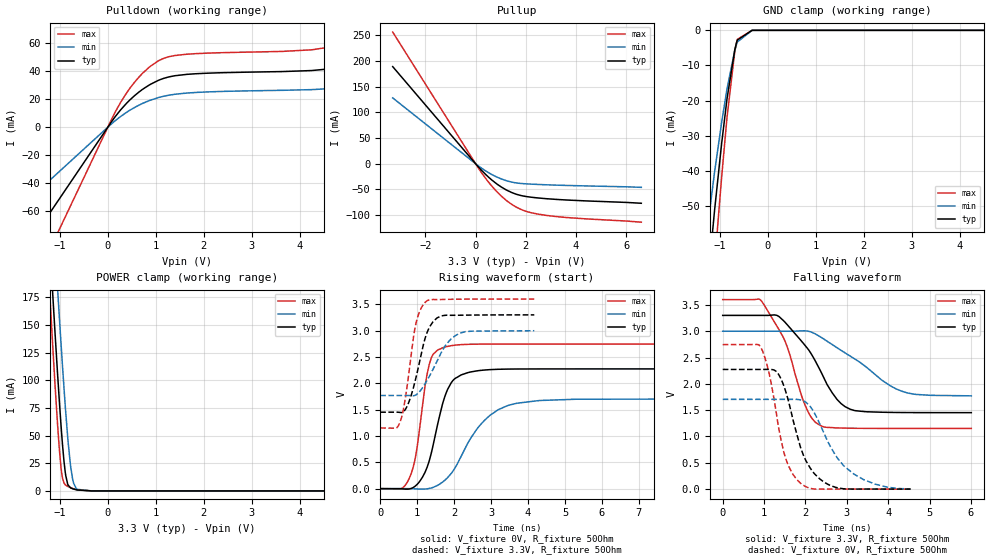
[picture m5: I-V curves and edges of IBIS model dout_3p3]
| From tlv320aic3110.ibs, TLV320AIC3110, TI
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|   dout_3p3 Model
[Model]   dout_3p3
Model_type   3-state
Polarity   Non-Inverting
Vmeas = 1.65
Vref = 0
Cref = 10pF
Rref = 50
|   typ   min   max
|   (nom PVT)   (fast PVT)   (slow PVT)
C_comp   1.577e-12   1.531e-12   1.633e-12
| Where nom  PVT is Nominal Process, 3.3V, 27C
|   Fast PVT is Strong Process,  3.6V, -40C
|   Slow PVT is Weak Process,   3V, 125C
[Voltage Range]   3.3   3   3.6
|Junction Temperature
[Temperature Range]   27   125   -40
[Pullup Reference]   3.3   3   3.6
[Pulldown Reference]   0   0   0
[Power Clamp Reference]   3.3   3   3.6
[GND Clamp Reference]   0   0   0
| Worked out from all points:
|   slope of the pulldown table from 0 to 0.495 V, typ, clamps not added: 24.1 ohm
|   slope of the pullup table from 0 to 0.495 V, typ, clamps not added: 19.6 ohm
|   POWER clamp passes 1 mA (typ) near -0.65 V on its own axis
|   falling waveform, V_fixture 3.3V, R_fixture 50Ohm: 20-80 % time 881ps typ, 1.32ns min, 668ps max; typ from 3.3 V to 1.45 V
|   rising waveform, V_fixture 0V, R_fixture 50Ohm: 20-80 % time 494ps typ, 951ps min, 336ps max; typ from 0 V to 2.27 V
|   rising waveform, V_fixture 3.3V, R_fixture 50Ohm: 20-80 % time 392ps typ, 569ps min, 297ps max; typ from 1.45 V to 3.3 V
|   falling waveform, V_fixture 0V, R_fixture 50Ohm: 20-80 % time 536ps typ, 810ps min, 414ps max; typ from 2.27 V to 0 V
[Pulldown]
|   Voltage   I(typ)   I(min)   I(max)
-3.3V     -167.2mA   -103.4mA   -238.3mA
-142.8mV  -7.234mA   -4.473mA   -10.31mA
153mV     7.459mA    4.581mA    10.75mA
462mV     19.5mA     12.14mA    27.88mA
855mV     29.92mA    18.83mA    42.57mA
1.164V    34.82mA    22.06mA    49.12mA
1.827V    38.11mA    24.74mA    52.46mA
4.713V    41.96mA    27.72mA    57.69mA
5.409V    48.18mA    31.48mA    67.5mA
5.732V    53.68mA    34.86mA    76.04mA
6.33V     70.28mA    45.19mA    101.5mA
6.6V      81.15mA    52.04mA    118mA
[GND Clamp]
|   Voltage   I(typ)   I(min)   I(max)
-3.3V     -1.792A    -1.545A    -1.979A
-1.482V   -105.6mA   -80.57mA   -134.7mA
-1.119V   -52.39mA   -41.19mA   -68.09mA
-1.104V   -50.35mA   -39.68mA   -65.46mA
-966.9mV  -32.64mA   -26.54mA   -42.36mA
-851.4mV  -19.49mA   -16.66mA   -24.78mA
-690mV    -5.595mA   -5.789mA   -6.089mA
-660mV    -3.881mA   -4.332mA   -3.916mA
-636mV    -2.764mA   -3.329mA   -2.575mA
-330mV    -1.038uA   -9.723uA   -110.9nA
6.6V      0A         0A         0A
[Pullup]
|   Voltage   I(typ)   I(min)   I(max)
-3.3V     189.2mA    128.2mA    256.5mA
181.2mV   -9.972mA   -6.723mA   -13.56mA
492mV     -25.14mA   -16.79mA   -34.41mA
786mV     -37.23mA   -24.59mA   -51.33mA
1.275V    -52.45mA   -33.81mA   -73.46mA
1.566V    -58.58mA   -37.05mA   -83.09mA
1.881V    -62.82mA   -38.83mA   -90.58mA
2.201V    -65.24mA   -39.78mA   -95.4mA
2.798V    -68.14mA   -41.09mA   -100.7mA
3.633V    -70.8mA    -42.41mA   -105mA
6.6V      -77.12mA   -46.09mA   -114mA
[POWER Clamp]
|   Voltage   I(typ)   I(min)   I(max)
-3.3V     1.931A     1.974A     1.932A
-1.264V   264.5mA    341.7mA    219.4mA
-1.151V   179.2mA    257.2mA    132.4mA
-1.05V    107.1mA    184.3mA    61.24mA
-1.013V   82.4mA     158.5mA    38.91mA
-960mV    49.9mA     122.5mA    15.45mA
-877.8mV  13.88mA    71.03mA    5.205mA
-777mV    2.767mA    22.45mA    2.971mA
-732mV    1.91mA     10.11mA    2.22mA
-633mV    837.8uA    1.394mA    916.8uA
-330mV    1.475uA    5.07uA     328.5nA
6.6V      0A         0A         0A
[Ramp]
R_load = 50
|   typ   min   max
dV/dt_r   1.36424/4.91213e-10   1.02269/9.48162e-10   1.64702/3.34704e-10
dV/dt_f   1.10914/8.80692e-10   0.738686/1.31383e-09   1.46874/6.6798e-10
[Falling Waveform]
V_fixture = 3.3V
V_fixture_min = 3V
V_fixture_max = 3.6V
R_fixture = 50Ohm
|   Time   V(typ)   V(min)   V(max)
0s        3.3V       3V         3.6V
939ps     3.3V       3V         3.572V
1.473ns   3.198V     3V         2.871V
1.99ns    2.73V      3.007V     1.597V
2.16ns    2.543V     2.977V     1.341V
2.37ns    2.236V     2.888V     1.205V
2.765ns   1.702V     2.685V     1.162V
3.187ns   1.492V     2.475V     1.156V
4.347ns   1.455V     1.855V     1.153V
6.009ns   1.452V     1.772V     1.152V
[Rising Waveform]
V_fixture = 0V
V_fixture_min = 0V
V_fixture_max = 0V
R_fixture = 50Ohm
|   Time   V(typ)   V(min)   V(max)
0s        1.342nV    19.15nV    904.1pV
559ps     -1.168mV   -14.88uV   -4.492mV
788ps     -6.16mV    593.2uV    200.2mV
966ps     59.54mV    -4.763mV   648.2mV
1.326ns   528.1mV    3.269mV    2.359V
1.7ns     1.643V     131.4mV    2.677V
2.184ns   2.158V     607mV      2.734V
2.853ns   2.254V     1.318V     2.744V
3.702ns   2.272V     1.622V     2.745V
12ns      2.274V     1.704V     2.745V
[Rising Waveform]
V_fixture = 3.3V
V_fixture_min = 3V
V_fixture_max = 3.6V
R_fixture = 50Ohm
|   Time   V(typ)   V(min)   V(max)
0s        1.451V     1.769V     1.152V
423ps     1.452V     1.769V     1.147V
538ps     1.447V     1.769V     1.267V
733ps     1.574V     1.769V     1.977V
966ps     2.107V     1.78V      3.139V
1.263ns   2.957V     2.051V     3.566V
1.537ns   3.242V     2.42V      3.591V
1.805ns   3.293V     2.756V     3.594V
2.166ns   3.293V     2.955V     3.598V
4.17ns    3.3V       2.998V     3.6V
[Falling Waveform]
V_fixture = 0V
V_fixture_min = 0V
V_fixture_max = 0V
R_fixture = 50Ohm
|   Time   V(typ)   V(min)   V(max)
0s        2.274V     1.705V     2.745V
919ps     2.274V     1.705V     2.699V
1.128ns   2.274V     1.705V     2.177V
1.38ns    2.139V     1.704V     1.051V
1.584ns   1.689V     1.705V     452.8mV
1.882ns   789.6mV    1.695V     111.2mV
2.343ns   195.3mV    1.243V     1.009mV
2.735ns   32.27mV    633.9mV    1.11mV
3.162ns   -128uV     289.8mV    495.2uV
4.54ns    317.1uV    2.361mV    58.94uV
